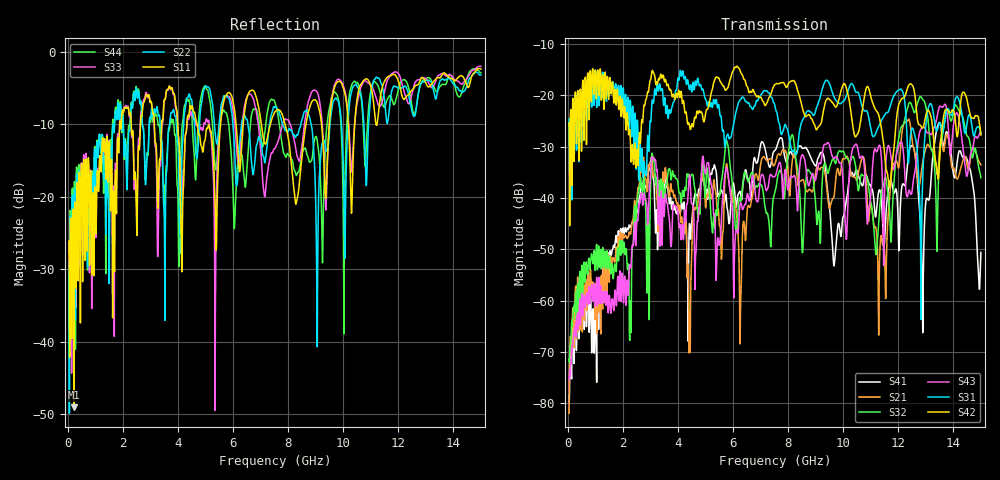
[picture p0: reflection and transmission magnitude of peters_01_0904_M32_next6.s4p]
# MHZ S RI R 50.00
! FREQ  S11  S12  S13  S14
!  S21  S22  S23  S24
!  S31  S32  S33  S34
!  S41  S42  S43  S44
!  REAL  IMAG  REAL  IMAG  REAL  IMAG  REAL  IMAG
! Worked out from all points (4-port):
!   1496 points, 50 MHz to 15 GHz, reference 50 ohm
!   strongest paths, dB at 50 MHz, 3.79 GHz, 7.53 GHz, 11.27 GHz, 15 GHz:
!     S42: -25.4, -20.2, -17.9, -23.5, -27.7
!     S31: -24.7, -22.3, -22.2, -26.3, -27.7
!     S43: -75.3, -45.9, -35.8, -30.3, -27.2
!     S32: -71.4, -35.0, -38.7, -46.5, -36.1
!     S21: -81.9, -38.7, -33.3, -56.9, -33.6
!     S41: -79.8, -41.5, -30.7, -39.3, -50.6
!   lowest |S11| = -49.1 dB at 220 MHz (marker M1), VSWR 1.01, Z = 49.7 + j0.161 ohm
!   |S11| at or under -10 dB: start of sweep to 1.888 GHz; 4.695 GHz to 5.548 GHz (853.5 MHz wide, 16.7 % of centre); 7.887 GHz to 8.649 GHz (761.8 MHz wide, 9.21 % of centre)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
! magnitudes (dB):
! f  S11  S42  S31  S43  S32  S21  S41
! 50 MHz  -26.1  -25.4  -24.7  -75.3  -71.4  -81.9  -79.8
! 220 MHz  -49.1  -27.1  -25.4  -66.7  -61.2  -65.1  -69.1
! 7.72 GHz  -8.1  -17.6  -26.7  -33.3  -34.6  -31.7  -28.3
! 11.2 GHz  -10.1  -23.0  -27.2  -30.9  -51.0  -46.2  -43.0
! 12.88 GHz  -3.5  -26.4  -37.6  -26.4  -20.7  -33.4  -62.0
! 13.49 GHz  -3.6  -33.6  -25.4  -22.3  -33.2  -31.1  -25.3
! 15 GHz  -2.4  -27.7  -27.7  -27.2  -36.1  -33.6  -50.6
